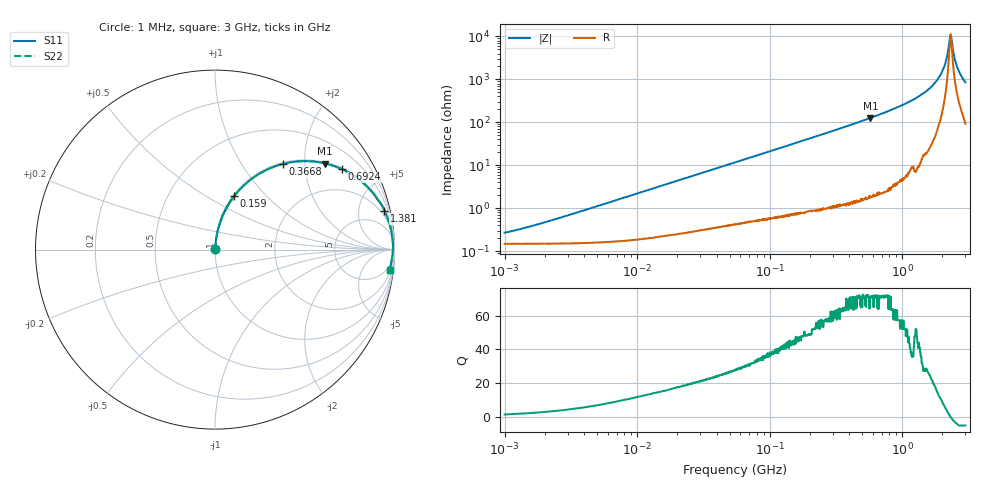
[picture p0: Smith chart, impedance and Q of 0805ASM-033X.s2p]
!s-Parameter Generated by FASTRON Sdn. Bhd.
!FASTRON P/N : 0805ASM-033X
!Keysight Technologies: E4991B_MY54100416_A.01.15
!Date: Fri Jun 19 14:48:24 2026
!Version  :Rev00  Fri Jun 19 14:48:24 2026
!Data & Calibration Information:
!Freq  S11  S21  S12  S22
!PortZ  Port1:50+j0  Port2:50+j0
!When reading reference impedance value at option line is always used.
! Remarks : This data is being provided solely for informational purposes.
# Hz S dB R 50
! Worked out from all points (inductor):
!   1601 points, 1 MHz to 3 GHz, reference 50 ohm
!   read as one part in series: L = 35.2 nH near 2.025 MHz
!   highest Q = 71.8 at 575.4 MHz (marker M1), where L = 35 nH
!   self-resonance near 2.313 GHz
!   S11 on the Smith chart (normalised r, x): 1 MHz: 1.00, +0.00; 159 MHz: 1.01, +0.67; 366.8 MHz: 1.02, +1.56; 692.4 MHz: 1.05, +3.12; 1.381 GHz: 1.24, +8.67; 3 GHz: 3, -17
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1000000  -51.50 56.2  -0.01 -0.1  -0.01 -0.1  -51.50 56.2
3804036  -41.40 79.2  -0.01 -0.5  -0.01 -0.5  -41.40 79.2
1.447069e7  -30.00 84.3  -0.02 -1.8  -0.02 -1.8  -30.00 84.3
5.504702e7  -18.70 81.3  -0.09 -6.6  -0.09 -6.6  -18.70 81.3
1.590202e8  -10.00 70.4  -0.52 -18.3  -0.52 -18.3  -10.00 70.4
2.083556e8  -8.00 65.4  -0.82 -23.5  -0.82 -23.5  -8.00 65.4
3.667557e8  -4.29 51.5  -2.13 -37.6  -2.13 -37.6  -4.29 51.5
5.753936e8  -2.17 38.0  -4.21 -51.2  -4.21 -51.2  -2.17 38.0
6.924261e8  -1.55 32.4  -5.43 -56.8  -5.43 -56.8  -1.55 32.4
7.925923e8  -1.17 28.3  -6.48 -60.9  -6.48 -60.9  -1.17 28.3
1.381259e9  -0.28 12.9  -13.00 -75.5  -13.00 -75.5  -0.28 12.9
1.67054e9  -0.15 8.2  -16.90 -79.2  -16.90 -79.2  -0.15 8.2
1.941122e9  -0.09 4.5  -22.10 -80.4  -22.10 -80.4  -0.09 4.5
2.102926e9  -0.07 2.5  -27.00 -77.7  -27.00 -77.7  -0.07 2.5
2.167021e9  -0.07 1.8  -30.00 -73.9  -30.00 -73.9  -0.07 1.8
2.255531e9  -0.07 0.7  -36.20 -56.3  -36.20 -56.3  -0.07 0.7
2.312676e9  -0.08 0.1  -40.90 -12.3  -40.90 -12.3  -0.08 0.1
2.383164e9  -0.08 -0.6  -36.60 49.5  -36.60 49.5  -0.08 -0.6
2.505452e9  -0.10 -1.9  -29.10 70.1  -29.10 70.1  -0.10 -1.9
2.620866e9  -0.12 -3.0  -25.30 74.4  -25.30 74.4  -0.12 -3.0
2.811057e9  -0.14 -4.8  -21.40 76.4  -21.40 76.4  -0.14 -4.8
3e9  -0.17 -6.6  -18.80 77.2  -18.80 77.2  -0.17 -6.6
